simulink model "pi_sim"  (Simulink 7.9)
settings: Solver=FixedStepDiscrete  SolverMode=SingleTasking  StartTime=0.0  StopTime=500  FixedStep=1  RelTol=1e-3  AbsTol=1e-6
PreLoadFcn:
  | init_exercise_4
InitFcn:
  | init_exercise_4
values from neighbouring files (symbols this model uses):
  a = 1    [init_exercise_4.m]    (also in noncausalfilter.m = [a(1,Na:end) zeros(1,Na-1)]; system_postloadfcn.m)
  am = 0.5    [init_exercise_4.m]    (also in system_postloadfcn.m)
  b = 1    [init_exercise_4.m]    (also in system_postloadfcn.m)
  w = 0.1    [init_exercise_4.m]    (also in system_postloadfcn.m)
libraries: labmvlib x2

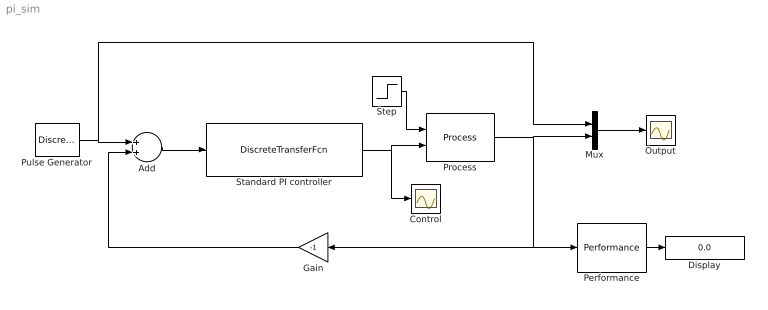
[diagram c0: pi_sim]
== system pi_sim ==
  Add : Sum
  Control : Scope
  Display : Display
  Gain : Gain  Gain=-1  SampleTime=1
  Mux : Mux  Inputs=2
  Output : Scope
  Performance : labmvlib/Performance
  Process : labmvlib/Process
  Pulse Generator : DiscretePulseGenerator  PulseType=Time based  Amplitude=5  Period=100  PulseWidth=50
  Standard PI controller : DiscreteTransferFcn  Numerator=[(1+a-am)/b -a/b]  Denominator=[1 -1]  SampleTime=1  a0EqualsOne=on
  Step : Step  Time=250  Before=w  After=10*w  SampleTime=1
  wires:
  Performance/1 -> Display/1
  Step/1 -> Process/1
  Standard PI controller/1 -> Control/1, Process/2
  Add/1 -> Standard PI controller/1
  Gain/1 -> Add/2
  Mux/1 -> Output/1
  Process/1 -> Mux/2, Performance/1, Gain/1
  Pulse Generator/1 -> Add/1, Mux/1
